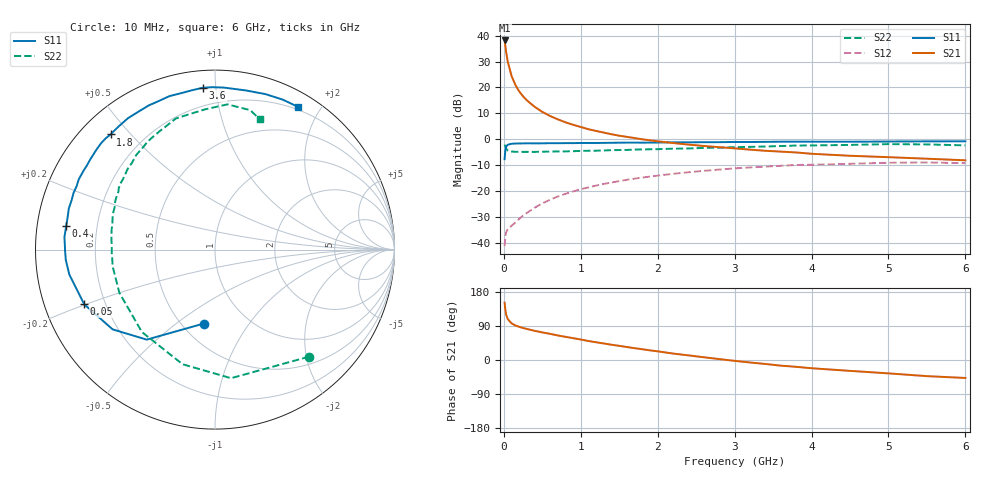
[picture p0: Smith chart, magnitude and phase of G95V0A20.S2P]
! SIEMENS Small Signal Semiconductors
! BFG235
! Si NPN RF Bipolar Junction Transistor in SOT223
! VCE = 5 V  IC = 200 mA
! Common Emitter S-Parameters:  July  1994
# GHz  S  MA  R  50
!  f  S11  S21  S12  S22
! GHz  MAG  ANG  MAG  ANG  MAG  ANG  MAG  ANG
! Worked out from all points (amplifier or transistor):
!   40 points, 10 MHz to 6 GHz, reference 50 ohm
!   highest |S21| = 38.1 dB at 10 MHz (marker M1)
!   |S21| within 3 dB of that: start of sweep to 23.5 MHz
!   unconditionally stable (mu >= 1): 430.2 MHz to 1.511 GHz
!   at 200 MHz: K = 0.83, MSG = 24.5 dB, |S12| = -30.5 dB
!   at 1.5 GHz: K = 1.00, MAG = 8.5 dB, |S12| = -16.0 dB
!   at 6 GHz: K = 0.90, MSG = 0.5 dB, |S12| = -9.1 dB
!   S11 on the Smith chart (normalised r, x): 10 MHz: 0.64, -0.63; 50 MHz: 0.12, -0.20; 400 MHz: 0.09, +0.08; 1.8 GHz: 0.09, +0.44; 3.6 GHz: 0.09, +0.92; 6 GHz: 0.17, +1.73
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0.01  0.4167 -98.6  80.4 151.2  0.0088 61.2  0.7939 -48.7
0.02  0.6297 -127.2  62.23 131.9  0.0138 47.4  0.7221 -82.9
0.03  0.7232 -142.1  48.24 120.2  0.0162 40.5  0.6637 -105.8
0.05  0.7898 -157.3  31.81 108.1  0.0185 34.0  0.6137 -131.6
0.1  0.8235 -170.3  16.71 96.8  0.0218 39.0  0.5847 -155.7
0.15  0.8334 -176.1  11.21 91.1  0.025 45.5  0.5758 -165.7
0.2  0.8351 -179.5  8.386 87.5  0.0297 50.5  0.5782 -170.9
0.25  0.8379 177.5  6.752 84.4  0.0341 54.0  0.5748 -174.6
0.3  0.8418 175.3  5.637 81.9  0.0384 56.6  0.5759 -177.8
0.4  0.8394 171.1  4.244 77.0  0.0483 59.8  0.5749 178.1
0.5  0.8407 167.5  3.387 72.8  0.0587 60.7  0.5796 174.7
0.7  0.8449 161.0  2.441 64.8  0.0793 60.9  0.5869 168.8
0.9  0.8481 155.4  1.912 57.6  0.0996 58.7  0.5936 164.2
1.1  0.8542 149.0  1.571 50.1  0.1195 55.9  0.6041 159.4
1.4  0.8603 142.0  1.258 40.3  0.1479 50.9  0.6201 153.2
1.8  0.8662 132.2  1.004 28.4  0.1841 43.8  0.6427 145.1
2.2  0.8781 123.5  0.852 17.0  0.2174 36.1  0.6627 137.2
3.2  0.8917 102.3  0.636 -6.6  0.2885 16.7  0.7177 118.6
3.6  0.9042 94.3  0.582 -14.9  0.3108 8.3  0.7447 110.3
4.5  0.9033 78.9  0.484 -28.7  0.3391 -7.9  0.7832 94.1
5.5  0.9168 65.8  0.425 -42.6  0.3595 -26.0  0.8013 75.8
6  0.9203 59.7  0.396 -47.4  0.3493 -32.8  0.768 71.1
